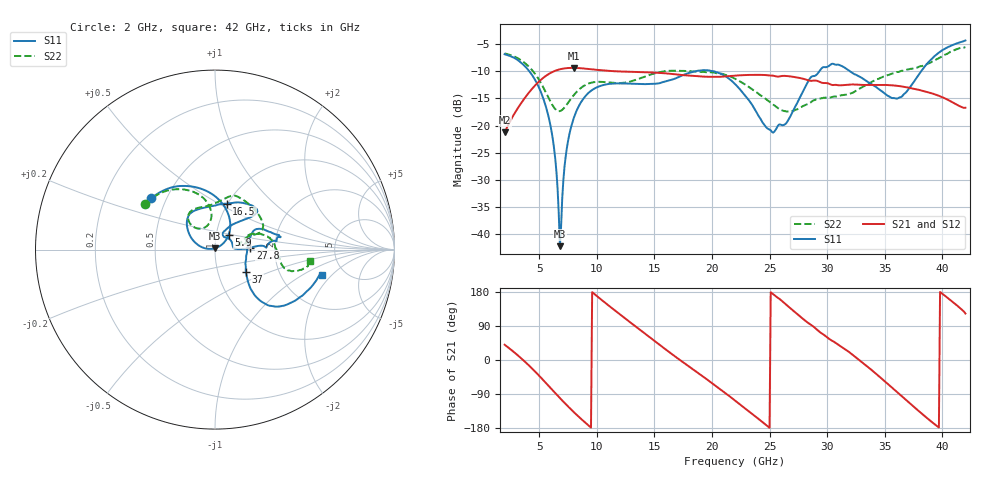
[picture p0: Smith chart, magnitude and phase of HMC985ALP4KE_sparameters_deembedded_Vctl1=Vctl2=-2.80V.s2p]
!s2p File: Measurements: S11, S21, S12, S22
# GHz S dB R 50.0
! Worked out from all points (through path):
!   401 points, 2 GHz to 42 GHz, reference 50 ohm
!   highest |S21| = -9.34 dB at 8 GHz (marker M1); lowest = -21.3 dB at 2 GHz (marker M2)
!   lowest |S11| = -42.3 dB at 6.8 GHz (marker M3), VSWR 1.02, Z = 50 + j0.769 ohm
!   |S11| at or under -10 dB: 4.156 GHz to 18.51 GHz (14.35 GHz wide, 127 % of centre); 20.21 GHz to 29.31 GHz (9.099 GHz wide, 36.7 % of centre); 31.99 GHz to 38.15 GHz (6.153 GHz wide, 17.5 % of centre)
!   |S22| runs from -17.4 to -5.5 dB; largest |S21 - S12| = 0.0004
!   S11 on the Smith chart (normalised r, x): 2 GHz: 0.41, +0.30; 5.9 GHz: 1.15, +0.19; 16.5 GHz: 0.99, +0.55; 27.8 GHz: 1.49, +0.03; 37 GHz: 1.36, -0.35; 42 GHz: 3.39, -1.54
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2  -6.82 141.1  -21.26 40.4  -21.27 40.4  -6.67 146.8
4.4  -10.71 88.5  -13.16 -23.0  -13.17 -23.0  -9.79 107.1
5.9  -19.17 46.7  -10.38 -71.0  -10.39 -71.0  -15.22 97.2
6.3  -24.32 37.7  -9.96 -84.1  -9.96 -84.1  -16.69 104.0
6.8  -42.28 89.6  -9.60 -100.4  -9.61 -100.4  -17.32 118.0
7.4  -24.22 171.7  -9.39 -119.3  -9.39 -119.3  -16.13 130.7
8  -18.63 160.5  -9.34 -137.3  -9.35 -137.3  -14.40 134.0
8.7  -15.46 148.7  -9.43 -157.1  -9.43 -157.1  -12.93 131.4
12.3  -12.20 118.7  -10.03 113.6  -10.03 113.5  -12.11 97.6
15.4  -12.19 89.6  -10.28 41.2  -10.28 41.2  -10.15 73.7
16.5  -11.55 75.6  -10.45 16.0  -10.45 16.0  -9.88 68.5
19.5  -9.79 44.6  -10.98 -49.7  -10.99 -49.7  -10.15 41.3
22  -12.31 44.7  -10.78 -106.9  -10.79 -106.9  -11.35 20.9
25.2  -21.17 56.9  -10.77 176.3  -10.77 176.3  -15.95 17.5
27.8  -14.11 2.9  -11.29 111.1  -11.29 111.1  -16.53 10.1
28.7  -10.90 2.2  -11.73 90.6  -11.74 90.6  -15.51 11.1
30.5  -8.58 10.8  -12.52 49.7  -12.53 49.6  -14.68 18.3
32.4  -10.54 21.8  -12.42 9.1  -12.43 9.1  -13.73 23.4
35.4  -14.64 6.5  -12.53 -66.8  -12.53 -66.8  -10.60 14.8
37  -13.46 -35.8  -12.97 -109.5  -12.98 -109.5  -9.64 6.3
39.6  -6.71 -43.4  -14.42 -175.9  -14.43 -175.9  -7.67 -15.5
42  -4.28 -13.4  -16.71 122.6  -16.72 122.6  -5.49 -7.0
